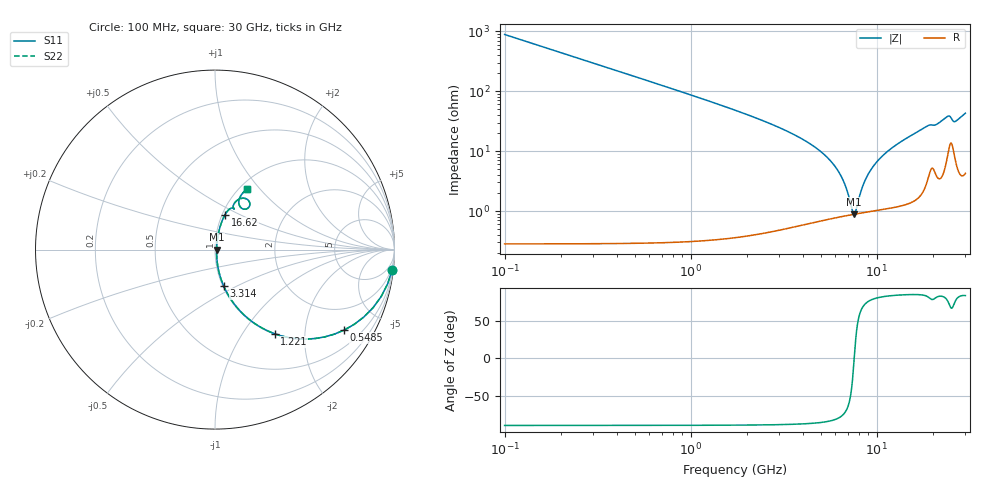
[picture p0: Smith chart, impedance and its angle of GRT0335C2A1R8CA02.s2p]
!Murata Part Number: GRT0335C2A1R8CA02
!These Parameters are Measured in Series Mode Connection
!Data Generated on Jun 19, 2026
!  o--ll--o
!Port1  Port2
!  o------o
!Operation Temp=25[degC], DC Bias Voltage=0[V]
!Freq. Start=100[MHz] Stop=30[GHz] 401[Steps]
# Hz S RI R 50
!Freq.(Hz) S11(Real) S11(Imag) S21(Real) S21(Imag) S12(Real) S12(Imag) S22(Real) S22(Imag)
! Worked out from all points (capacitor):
!   401 points, 100 MHz to 30 GHz, reference 50 ohm
!   read as one part in series: C = 1.8 pF near 249.5 MHz
!   lowest |Z| = 885 mohm at 7.575 GHz (marker M1)
!   series resonance near 7.574 GHz, so ESL is about 250 pH
!   S11 on the Smith chart (normalised r, x): 100 MHz: 1, -18; 548.5 MHz: 1.01, -3.21; 1.221 GHz: 1.01, -1.41; 3.314 GHz: 1.01, -0.43; 16.62 GHz: 1.03, +0.42; 30 GHz: 1.09, +0.85
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1e8  0.9873 -0.1117  0.0127 0.1117  0.0127 0.1117  0.9873 -0.1117
3.2425e8  0.8808 -0.3235  0.1192 0.3235  0.1192 0.3235  0.8808 -0.3235
5.485e8  0.7195 -0.4483  0.2805 0.4483  0.2805 0.4483  0.7195 -0.4483
8.475e8  0.5145 -0.4983  0.4855 0.4983  0.4855 0.4983  0.5145 -0.4983
1.22125e9  0.3322 -0.4687  0.6678 0.4687  0.6678 0.4687  0.3322 -0.4687
2.0435e9  0.1402 -0.3424  0.8598 0.3424  0.8598 0.3424  0.1402 -0.3424
3.31425e9  0.0483 -0.2027  0.9517 0.2027  0.9517 0.2027  0.0483 -0.2027
5.10825e9  0.0153 -0.0911  0.9847 0.0911  0.9847 0.0911  0.0153 -0.0911
6.45375e9  0.00933 -0.0363  0.9907 0.0363  0.9907 0.0363  0.00933 -0.0363
6.90225e9  0.00877 -0.021  0.9912 0.021  0.9912 0.021  0.00877 -0.021
7.4255e9  0.0087 -0.00448  0.9913 0.00448  0.9913 0.00448  0.0087 -0.00448
7.575e9  0.00877 2.41e-05  0.9912 -2.41e-05  0.9912 -2.41e-05  0.00877 2.41e-05
8.69625e9  0.0104 0.0313  0.9896 -0.0313  0.9896 -0.0313  0.0104 0.0313
1.01165e10  0.0146 0.066  0.9854 -0.066  0.9854 -0.066  0.0146 0.066
1.213475e10  0.0235 0.1097  0.9765 -0.1097  0.9765 -0.1097  0.0235 0.1097
1.505e10  0.0422 0.1663  0.9578 -0.1663  0.9578 -0.1663  0.0422 0.1663
1.661975e10  0.0564 0.1954  0.9436 -0.1954  0.9436 -0.1954  0.0564 0.1954
2.005825e10  0.1063 0.2264  0.8937 -0.2264  0.8937 -0.2264  0.1063 0.2264
2.38705e10  0.1661 0.2854  0.8339 -0.2854  0.8339 -0.2854  0.1661 0.2854
2.50665e10  0.1908 0.2394  0.8092 -0.2394  0.8092 -0.2394  0.1908 0.2394
2.618775e10  0.1425 0.2358  0.8575 -0.2358  0.8575 -0.2358  0.1425 0.2358
3e10  0.1787 0.3365  0.8213 -0.3365  0.8213 -0.3365  0.1787 0.3365
